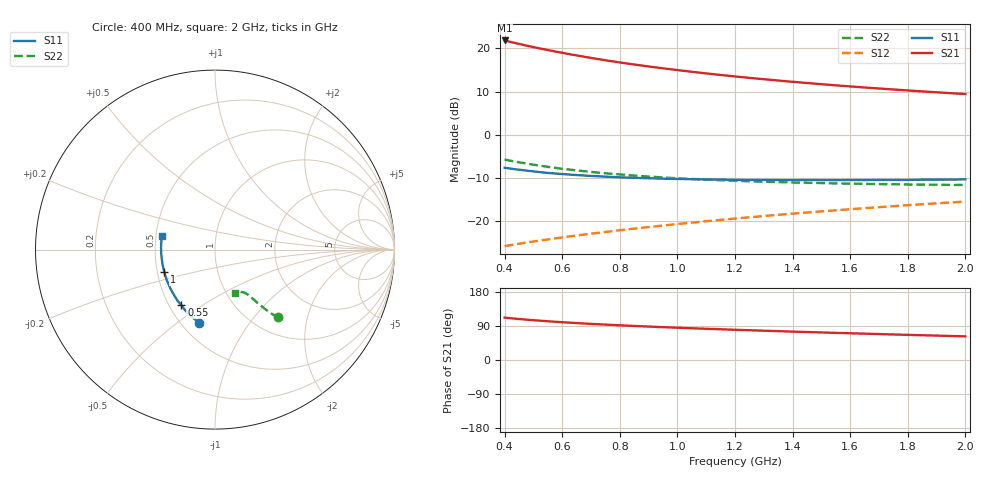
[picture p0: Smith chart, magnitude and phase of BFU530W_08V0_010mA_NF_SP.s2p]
! Filename:  P:\Prog\Test\Noise\ATS_data\Testdata_Net\06 Compressed Noise after Statistics\BFU530W_APM2013_09_A05_08p0V_010mA_NF_CM01_D.sf
! Date/Time: Tue 26/Mar/2013 18:06:03
! BFU530W_APM2013_09_A05_08p0V_1to25mA_NF_CM01_Bias6_R.sf
! Noise Parameter Data File
! BFU530W_APM2013_09_A05_08p0V_1to25mA_NF_CM01
! Date/time: Thu Mar 21 21:44:48 2013
! VAR V_out= 8.000000
! VAR I_out= 10.000000
! VAR V_in= 0.815100
! VAR I_in= 0.100810
! Device data file deembeded for feedlines and parallel
! Original file: \06 Compressed Noise after Statistics\BFU530W_APM2013_09_A05_08p0V_010mA_NF_CM01_R.sf
! Feed-files: PR019V01_070313_Feed1.s2p, PR019V01_070313_Feed2.s2p
! Parallel-file: PR019V01_070313_Par.s2p
# MHz S MA R 50
!  Freq-MHz  S11-mag  S11-arg  S21-mag  S21-arg  S12-mag  S12-arg  S22-mag  S22-arg
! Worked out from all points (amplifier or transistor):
!   37 points, 400 MHz to 2 GHz, reference 50 ohm
!   highest |S21| = 21.9 dB at 400 MHz (marker M1)
!   |S21| within 3 dB of that: start of sweep to 611.3 MHz
!   unconditionally stable (mu >= 1): 1.43 GHz to end of sweep
!   at 500 MHz: K = 0.72, MSG = 22.5 dB, |S12| = -24.7 dB
!   at 1.1 GHz: K = 0.96, MSG = 17.1 dB, |S12| = -20.0 dB
!   at 2 GHz: K = 1.02, MAG = 11.7 dB, |S12| = -15.4 dB
!   lowest NFmin = 0.75 dB at 420 MHz
!   S11 on the Smith chart (normalised r, x): 400 MHz: 0.61, -0.60; 550 MHz: 0.58, -0.41; 1 GHz: 0.54, -0.15; 2 GHz: 0.54, +0.09
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400  0.4169 -102.3  12.39 111.8  0.0516 59.4  0.5178 -46.9
420  0.4077 -105.2  11.93 110.3  0.05298 59.3  0.5029 -47.6
433  0.4021 -107.0  11.65 109.4  0.05388 59.2  0.4935 -47.9
460  0.3922 -110.5  11.1 107.6  0.05574 59.4  0.4763 -48.5
500  0.3782 -115.6  10.38 105.0  0.05838 59.5  0.4522 -49.3
550  0.3628 -121.1  9.595 102.2  0.06178 59.9  0.4273 -50.0
600  0.3529 -126.3  8.91 99.7  0.06519 60.2  0.4057 -50.6
650  0.3431 -130.9  8.307 97.5  0.06855 60.6  0.3885 -51.1
700  0.3352 -135.4  7.779 95.3  0.07193 61.1  0.3732 -51.6
750  0.3291 -139.3  7.311 93.4  0.07535 61.5  0.3595 -51.9
800  0.3229 -143.1  6.897 91.6  0.07886 61.9  0.349 -52.4
850  0.319 -146.7  6.528 89.8  0.08235 62.2  0.3382 -52.6
950  0.3118 -152.9  5.897 86.7  0.08947 62.9  0.3222 -53.3
1000  0.3093 -155.9  5.625 85.2  0.09304 63.2  0.3147 -53.5
1100  0.3051 -161.2  5.149 82.4  0.1003 63.7  0.3041 -54.5
1200  0.3025 -166.1  4.751 79.8  0.1077 64.0  0.2953 -55.3
1250  0.3014 -168.4  4.572 78.5  0.1114 64.1  0.2908 -55.7
1350  0.3004 -172.5  4.26 76.1  0.119 64.3  0.285 -56.7
1500  0.3002 -178.4  3.863 72.7  0.1304 64.3  0.2773 -58.5
1650  0.3006 176.2  3.538 69.5  0.142 64.2  0.2714 -60.2
1750  0.3018 173.0  3.356 67.4  0.1499 64.1  0.2689 -61.5
2000  0.3063 165.5  2.971 62.4  0.1694 63.4  0.2638 -65.4
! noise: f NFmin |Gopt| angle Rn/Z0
400  0.7672  0.06035  143.1  0.0859
460  0.7775  0.07726  159.2  0.082
600  0.7801  0.06934  140.9  0.0896
800  0.8204  0.1087  155.7  0.0805
1000  0.8347  0.1228  159.8  0.0801
1200  0.9049  0.1421  164.9  0.0773
1400  0.908  0.1731  172.8  0.0723
1600  0.8998  0.1847  175.7  0.075
1800  0.9696  0.199  -177.2  0.0742
2000  0.9986  0.2118  -170.9  0.0782
